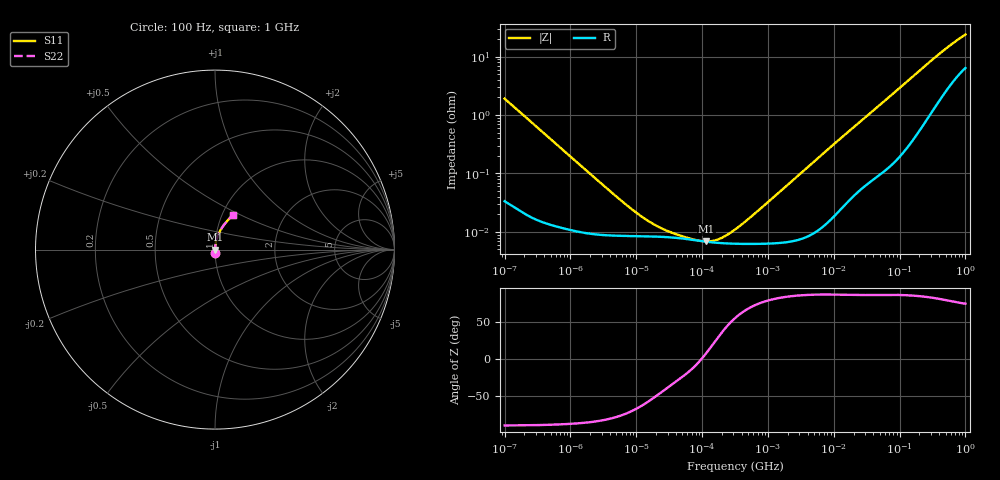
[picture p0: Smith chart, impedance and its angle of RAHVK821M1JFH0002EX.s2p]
! RAHVK821M1JFH0002EX  S-PARAMETER MODEL  (AEC-Q200 qualified)
! Model Generated by ELNA Corporation (http://www.ty-top.com)
! Version 1.0
! ELNA Control No.201028
! Copyright (c) 2020 ELNA CO.,LTD. All Rights Reserved.
! Products Name : CONDUCTIVE POLYMER HYBRID ALUMINUM ELECTROLYTIC CAPACITORS
! Characteristics :
!  Capacitance  :  820uF  ,  Rated voltage  :  6.3V
!  Operating Temp. Range  :  -55 to +125 degC  ,  Endurance  :  4000hr at 125 degC
!  Dimension D  :  10mm  ,  Dimension L  :  10mm
! Frequency Range : 100Hz - 1GHz
! External Node Assignments :
!  1  o---| |---o  2
# MHz S RI R 50
!Freq[MHz].  S11 Real  S11 Imag  S21 Real  S21 Imag  S12 Real  S12 Imag  S22 Real  S22 Imag
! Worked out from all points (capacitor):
!   401 points, 100 Hz to 1 GHz, reference 50 ohm
!   read as one part in series: C = 833 uF near 108 Hz
!   lowest |Z| = 6.86 mohm at 115.5 kHz (marker M1)
!   series resonance near 97.57 kHz, so ESL is about 3.2 nH
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0.0001  0.000697 -0.019  0.9993 0.019  0.9993 0.019  0.000697 -0.019
0.000133  0.000482 -0.0144  0.9995 0.0144  0.9995 0.0144  0.000482 -0.0144
0.001488  9.98e-05 -0.00131  0.9999 0.00131  0.9999 0.00131  9.98e-05 -0.00131
0.004597  8.65e-05 -0.000426  0.9999 0.000426  0.9999 0.000426  8.65e-05 -0.000426
0.008414  8.49e-05 -0.000233  0.9999 0.000233  0.9999 0.000233  8.49e-05 -0.000233
0.014207  8.4e-05 -0.000138  0.9999 0.000138  0.9999 0.000138  8.4e-05 -0.000138
0.022131  8.27e-05 -8.81e-05  0.9999 8.81e-05  0.9999 8.81e-05  8.27e-05 -8.81e-05
0.029343  8.14e-05 -6.56e-05  0.9999 6.56e-05  0.9999 6.56e-05  8.14e-05 -6.56e-05
0.034475  8.04e-05 -5.49e-05  0.9999 5.49e-05  0.9999 5.49e-05  8.04e-05 -5.49e-05
0.115478  6.8e-05 9.51e-06  0.9999 -9.51e-06  0.9999 -9.51e-06  6.8e-05 9.51e-06
0.258523  6.32e-05 6.91e-05  0.9999 -6.91e-05  0.9999 -6.91e-05  6.32e-05 6.91e-05
0.291743  6.29e-05 8.11e-05  0.9999 -8.11e-05  0.9999 -8.11e-05  6.29e-05 8.11e-05
0.316228  6.27e-05 8.99e-05  0.9999 -8.99e-05  0.9999 -8.99e-05  6.27e-05 8.99e-05
0.707946  6.24e-05 0.000221  0.9999 -0.000221  0.9999 -0.000221  6.24e-05 0.000221
4.704354  9.35e-05 0.0015  0.9999 -0.0015  0.9999 -0.0015  9.35e-05 0.0015
12.37371  0.000249 0.00387  0.9998 -0.00387  0.9998 -0.00387  0.000249 0.00387
69.9842  0.0017 0.0204  0.9983 -0.0204  0.9983 -0.0204  0.0017 0.0204
176.8072  0.00688 0.0501  0.9931 -0.0501  0.9931 -0.0501  0.00688 0.0501
380.1894  0.026 0.1003  0.974 -0.1003  0.974 -0.1003  0.026 0.1003
668.3439  0.0623 0.1531  0.9377 -0.1531  0.9377 -0.1531  0.0623 0.1531
922.5714  0.0933 0.1859  0.9067 -0.1859  0.9067 -0.1859  0.0933 0.1859
1000  0.102 0.1944  0.898 -0.1944  0.898 -0.1944  0.102 0.1944
